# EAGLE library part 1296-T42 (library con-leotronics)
1.27mm SINGLE ROW FEMALE SOCKET Source: http://www.leotronics.co.uk/Conexcon/Data%20Sheets/sec.%20A/1296ing.pdf
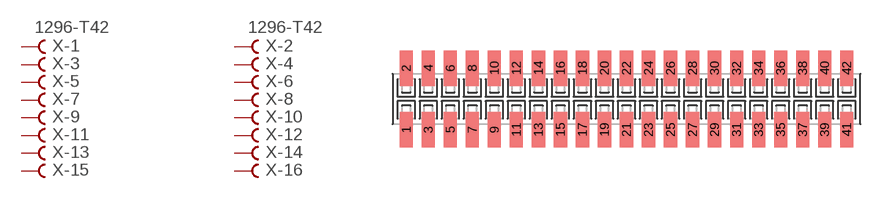
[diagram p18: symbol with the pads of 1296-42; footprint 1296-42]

Designator prefix X; gates -1=FVAL -2=FVAL -3=F -4=F -5=F -6=F -7=F -8=F -9=F -10=F -11=F -12=F -13=F -14=F -15=F -16=F -17=F -18=F -19=F -20=F -21=F -22=F -23=F -24=F -25=F -26=F -27=F -28=F -29=F -30=F -31=F -32=F -33=F -34=F -35=F -36=F -37=F -38=F -39=F -40=F -41=F -42=F

## 1296-T42 (OC_FARNELL: unknown; OC_NEWARK: unknown)  [1296-42]
1  -1:B  pas
2  -2:B  pas
3  -3:B  pas
4  -4:B  pas
5  -5:B  pas
6  -6:B  pas
7  -7:B  pas
8  -8:B  pas
9  -9:B  pas
10  -10:B  pas
11  -11:B  pas
12  -12:B  pas
13  -13:B  pas
14  -14:B  pas
15  -15:B  pas
16  -16:B  pas
17  -17:B  pas
18  -18:B  pas
19  -19:B  pas
20  -20:B  pas
21  -21:B  pas
22  -22:B  pas
23  -23:B  pas
24  -24:B  pas
25  -25:B  pas
26  -26:B  pas
27  -27:B  pas
28  -28:B  pas
29  -29:B  pas
30  -30:B  pas
31  -31:B  pas
32  -32:B  pas
33  -33:B  pas
34  -34:B  pas
35  -35:B  pas
36  -36:B  pas
37  -37:B  pas
38  -38:B  pas
39  -39:B  pas
40  -40:B  pas
41  -41:B  pas
42  -42:B  pas

## Footprint 1296-42 (pad centres in mm)
1.27mm SINGLE ROW FEMALE SOCKET Source: http://www.leotronics.co.uk/Conexcon/Data%20Sheets/sec.%20A/1296ing.pdf
smd 0.76 x 2.05: 1 -12.7,-1.78; 2 -12.7,1.78; 3 -11.43,-1.78; 4 -11.43,1.78; 5 -10.16,-1.78; 6 -10.16,1.78; 7 -8.89,-1.78; 8 -8.89,1.78; 9 -7.62,-1.78; 10 -7.62,1.78; 11 -6.35,-1.78; 12 -6.35,1.78; 13 -5.08,-1.78; 14 -5.08,1.78; 15 -3.81,-1.78; 16 -3.81,1.78; 17 -2.54,-1.78; 18 -2.54,1.78; 19 -1.27,-1.78; 20 -1.27,1.78; 21 0,-1.78; 22 0,1.78; 23 1.27,-1.78; 24 1.27,1.78; 25 2.54,-1.78; 26 2.54,1.78; 27 3.81,-1.78; 28 3.81,1.78; 29 5.08,-1.78; 30 5.08,1.78; 31 6.35,-1.78; 32 6.35,1.78; 33 7.62,-1.78; 34 7.62,1.78; 35 8.89,-1.78; 36 8.89,1.78; 37 10.16,-1.78; 38 10.16,1.78; 39 11.43,-1.78; 40 11.43,1.78; 41 12.7,-1.78; 42 12.7,1.78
